(* Logix 5000 AddOnInstructionDefinition export AMCI_SV160E2_Reset_Errors; software revision 20.03 *)

ADD_ON_INSTRUCTION AMCI_SV160E2_Reset_Errors   (* revision 1.0, vendor AMCI *)
// Revision note:
// 8/2019 Version 0 Initial release of SV160E2 Add On Instructions.
// 3/17/20 Version 1 replaced the generic EDS file with a more complete V1.6 EDS file.
VAR_IN_OUT
   AMCI_SV160E2_OUTPUT_DATA : _000A:SV160E2_9125ACD4:O:0; {required}
END_VAR
VAR
   command_data_block : INT[10];
        [0]   // Command Bits MSW
        [1]   // Command Bits LSW
        [2]   // Upper Target Position
        [3]   // Lower Target Position
        [4]   // Upper Programmed Speed
        [5]   // Lower Programmed Speed
END_VAR

ROUTINE Logic   (* ladder *)
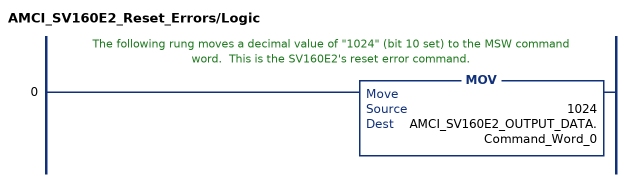
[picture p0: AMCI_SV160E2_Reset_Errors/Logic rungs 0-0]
   // The following rung moves a decimal value of "1024" (bit 10 set) to the MSW command word.  This is the SV160E2's reset error command.
   0: MOV(1024,AMCI_SV160E2_OUTPUT_DATA.Command_Word_0);
END_ROUTINE
END_ADD_ON_INSTRUCTION
